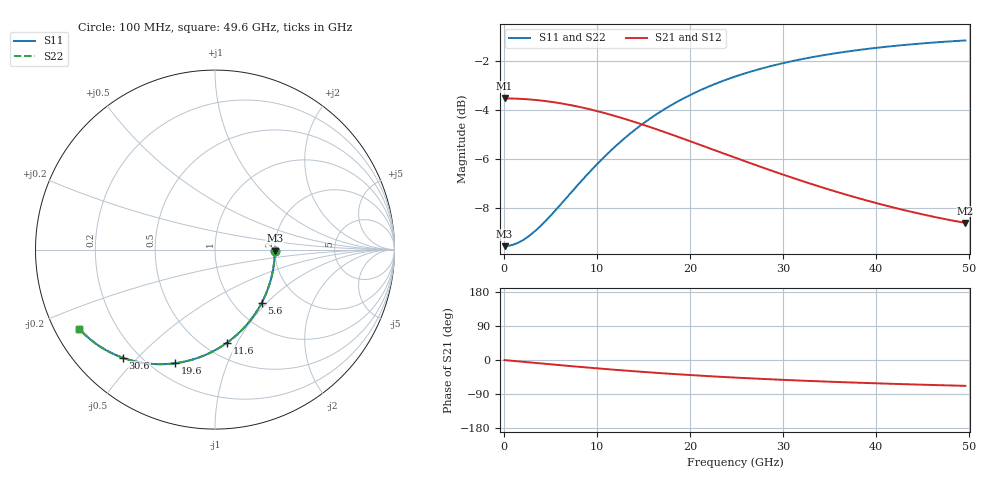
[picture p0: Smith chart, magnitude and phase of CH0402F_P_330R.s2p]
# GHz S RI R 330
! S-Parameters data
! Freq  reS11  imS11  reS21  imS21  reS12  imS12  reS22  imS22
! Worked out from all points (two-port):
!   100 points, 100 MHz to 49.6 GHz, reference 330 ohm
!   highest |S21| = -3.52 dB at 100 MHz (marker M1); lowest = -8.6 dB at 49.6 GHz (marker M2)
!   |S21| within 3 dB of the highest: start of sweep to 29.22 GHz
!   lowest |S11| = -9.5 dB at 100 MHz (marker M3), VSWR 2.00, Z = 660 - j8.38 ohm
!   |S11| at or under -10 dB: nowhere
!   |S22| runs from -9.5 to -1.2 dB; largest |S21 - S12| = 0
!   S11 on the Smith chart (normalised r, x): 100 MHz: 2.00, -0.03; 5.6 GHz: 1.32, -0.94; 11.6 GHz: 0.63, -0.91; 19.6 GHz: 0.29, -0.67; 30.6 GHz: 0.14, -0.46; 49.6 GHz: 0.07, -0.27
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0.1  0.3333 -0.00565  0.6667 -0.00265  0.6667 -0.00265  0.3333 -0.00565
1.1  0.3303 -0.062  0.6655 -0.0291  0.6655 -0.0291  0.3303 -0.062
2.6  0.3167 -0.1449  0.6603 -0.0683  0.6603 -0.0683  0.3167 -0.1449
4.1  0.2927 -0.2242  0.6511 -0.1063  0.6511 -0.1063  0.2927 -0.2242
5.6  0.2594 -0.2981  0.6382 -0.1426  0.6382 -0.1426  0.2594 -0.2981
7.1  0.2185 -0.3653  0.622 -0.1766  0.622 -0.1766  0.2185 -0.3653
8.6  0.1714 -0.4248  0.6029 -0.2079  0.6029 -0.2079  0.1714 -0.4248
10.1  0.12 -0.4763  0.5815 -0.2363  0.5815 -0.2363  0.12 -0.4763
11.6  0.0657 -0.5197  0.5585 -0.2616  0.5585 -0.2616  0.0657 -0.5197
14.1  -0.0272 -0.5748  0.5176 -0.2967  0.5176 -0.2967  -0.0272 -0.5748
16.6  -0.1188 -0.6107  0.4757 -0.3234  0.4757 -0.3234  -0.1188 -0.6107
18.1  -0.1716 -0.6244  0.4509 -0.3358  0.4509 -0.3358  -0.1716 -0.6244
19.6  -0.2222 -0.6331  0.4266 -0.3458  0.4266 -0.3458  -0.2222 -0.6331
22.1  -0.3009 -0.6384  0.3879 -0.3578  0.3879 -0.3578  -0.3009 -0.6384
25.1  -0.3852 -0.6332  0.3451 -0.366  0.3451 -0.366  -0.3852 -0.6332
27.6  -0.4471 -0.622  0.3129 -0.3689  0.3129 -0.3689  -0.4471 -0.622
30.6  -0.5121 -0.6031  0.2783 -0.3692  0.2783 -0.3692  -0.5121 -0.6031
33.1  -0.5591 -0.5843  0.2526 -0.3676  0.2526 -0.3676  -0.5591 -0.5843
37.1  -0.623 -0.551  0.217 -0.3629  0.217 -0.3629  -0.623 -0.551
41.6  -0.6807 -0.5115  0.1837 -0.3563  0.1837 -0.3563  -0.6807 -0.5115
45.6  -0.7219 -0.4761  0.159 -0.3504  0.159 -0.3504  -0.7219 -0.4761
49.6  -0.7556 -0.4412  0.1379 -0.3452  0.1379 -0.3452  -0.7556 -0.4412
